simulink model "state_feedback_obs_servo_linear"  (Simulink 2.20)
settings: Solver=ode1  StartTime=0.0  StopTime=999999  FixedStep=0.001  RelTol=1e-3  AbsTol=1e-6
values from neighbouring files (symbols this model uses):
  A = [ 0 1 ; 0 -13 ]    [design_state_feedback.m]    (also in design_state_feedback_obs.m)
  B = [ 0 ; 2.9 ]    [design_state_feedback.m]    (also in design_state_feedback_obs.m)
  C = [ 1 0 ]    [design_state_feedback.m]    (also in design_state_feedback_obs.m)
  hat_x0 = [ 0 ; 0 ]    [design_state_feedback_obs.m]
  K = place(A,B,[lambda1,lambda2])    [design_state_feedback.m]    (also in design_state_feedback_obs.m)
  kc = 1/(C*inv(B*K-A)*B)    [design_state_feedback.m]    (also in design_state_feedback_obs.m)
  L = (place(A',C',[mu1,mu2]))'    [design_state_feedback_obs.m]
libraries: simulink x5, winlib x3

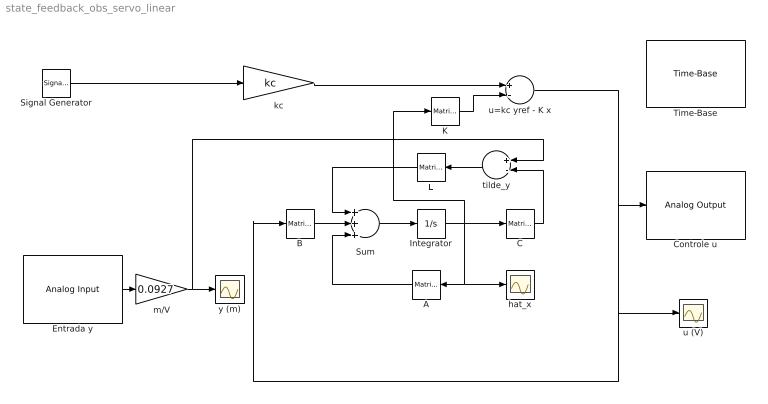
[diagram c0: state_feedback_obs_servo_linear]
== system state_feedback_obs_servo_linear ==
  A : simulink/Linear/Matrix Gain  Orientation=left  K=A
  B : simulink/Linear/Matrix Gain  K=B
  C : simulink/Linear/Matrix Gain  K=C
  Controle u : winlib/Quanser Consulting MultiQ Series/Analog Output  baseAddr=0x320  channels=[3]  initialOutputs=0  finalOutputs=0  sampleTime=str2num(get_param(bdroot, 'FixedStep'))
  Entrada y : winlib/Quanser Consulting MultiQ Series/Analog Input  baseAddr=0x320  channels=[1]  sampleTime=str2num(get_param(bdroot, 'FixedStep'))
  Integrator : Integrator  ExternalReset=none  InitialConditionSource=internal  InitialCondition=hat_x0  LimitOutput=off  UpperSaturationLimit=inf  LowerSaturationLimit=-inf  ShowSaturationPort=off  ShowStatePort=off  AbsoluteTolerance=auto
  K : simulink/Linear/Matrix Gain  K=K
  L : simulink/Linear/Matrix Gain  Orientation=left  K=L
  Signal Generator : SignalGenerator  WaveForm=square  Amplitude=0.05  Frequency=0.2  Units=Hertz
  Sum : Sum  Inputs=+++
  Time-Base : winlib/Quanser Consulting MultiQ Series/Time-Base  baseAddr=0x320  irqLevel=9  clockSource=1
  hat_x : Scope
  kc : Gain  Gain=kc
  m/V : Gain  Gain=0.0927
  tilde_y : Sum  Orientation=left  Inputs=+-
  u (V) : Scope
  u=kc yref - K x : Sum  Inputs=+-
  y (m) : Scope
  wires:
  u=kc yref - K x/1 -> Controle u/1, u (V)/1, B/1
  Signal Generator/1 -> kc/1
  kc/1 -> u=kc yref - K x/1
  Sum/1 -> Integrator/1
  A/1 -> Sum/3
  B/1 -> Sum/2
  Integrator/1 -> A/1, hat_x/1, C/1, K/1
  L/1 -> Sum/1
  C/1 -> tilde_y/2
  tilde_y/1 -> L/1
  K/1 -> u=kc yref - K x/2
  Entrada y/1 -> m/V/1
  m/V/1 -> y (m)/1, tilde_y/1
